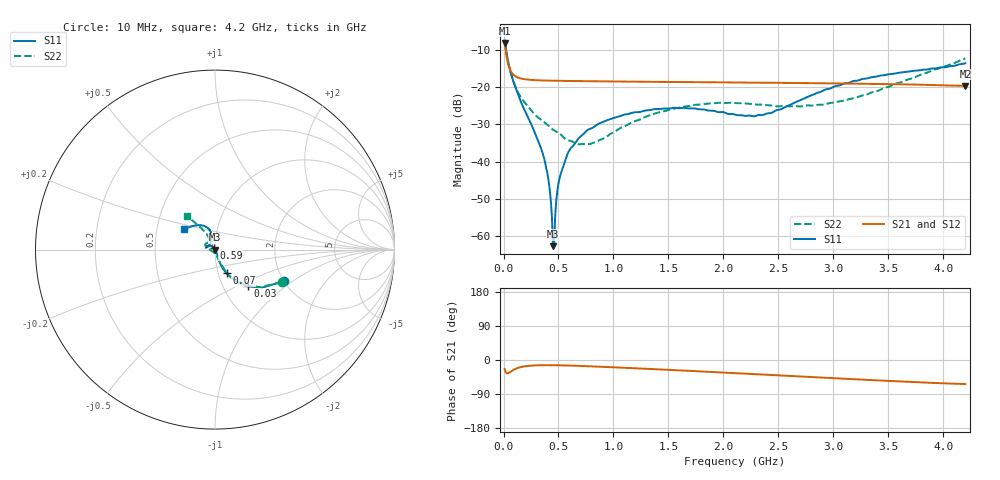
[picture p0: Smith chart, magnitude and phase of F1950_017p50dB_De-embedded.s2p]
! Integrated Device Technology
! Corporate Headquarters
! 6024 Silver Creek Valley Road
! San Jose, CA 95138  USA
! Phone:  1-408-284-8200
! Toll Free:  1-800-223-1366
! Webpage:  http://www.idt.com/
! Timing and RF Division
! 515 Groton Road, Suite 102
! Westford, MA 01886-6024
! Device:  F1950
! Description: 7-bit 0.25 dB Digital Step Attenuator
! Frequency:  150.0 -  4000.00 MHz
! Package:  4x4 mm Thin QFN Plastic Package: 24 pin
! Ports:  2 RF, 12 DC
!  Pin  1  = D0
!  Pin  2  = VDD
!  Pin  3  = Vmode
!  Pin  4  = GND
!  Pin  5  = RF1  =  Port 1
!  Pin  6  = GND
!  Pin  7  = GND
!  Pin  8  = GND
!  Pin  9  = GND
!  Pin 10  = GND
!  Pin 11  = GND
!  Pin 12  = GND
!  Pin 13  = GND
!  Pin 14  = RF2  =  Port 2
!  Pin 15  = GND
!  Pin 16  = LE
!  Pin 17  = CLK
!  Pin 18  = DATE
!  Pin 19  = D6
!  Pin 20  = D5
!  Pin 21  = D4
!  Pin 22  = D3
!  Pin 23  = D2
!  Pin 24  = D1
! State:  70
! Atten State:  17.50 dB
! Voltage:  +5.00 Volts
! Current:  Not Measured mA
! Data:  The device was measured on a the F195X evaluation board which has
!  individual transmission lines to the RF pins.  Data was collected
!  using a calibrated network analyzer.  The evaluation board was
!  de-embedded using a TRL calibration technique.
!  The reference plane is the edge of the package pin.
! Misc:  Board 2019
!  Action Tracker AT0250
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# GHz S dB R 50
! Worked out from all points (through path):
!   420 points, 10 MHz to 4.2 GHz, reference 50 ohm
!   highest |S21| = -8.20 dB at 10 MHz (marker M1); lowest = -19.7 dB at 4.2 GHz (marker M2)
!   group delay of S21, straight-line fit = 35.1 ps
!   lowest |S11| = -62.6 dB at 450 MHz (marker M3), VSWR 1.00, Z = 50.1 - j0.0332 ohm
!   |S11| at or under -10 dB: 22.86 MHz to end of sweep
!   |S22| runs from -35.4 to -7.7 dB; largest |S21 - S12| = 0.0002
!   S11 on the Smith chart (normalised r, x): 10 MHz: 1.99, -0.85; 30 MHz: 1.30, -0.57; 70 MHz: 1.10, -0.30; 590 MHz: 0.98, +0.02; 4.2 GHz: 0.69, +0.17
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0.01  -7.52 -24.8  -8.20 -23.7  -8.20 -23.7  -7.68 -26.0
0.03  -11.29 -48.2  -12.17 -35.3  -12.17 -35.3  -11.40 -48.2
0.07  -16.67 -63.9  -15.92 -29.8  -15.92 -29.8  -16.49 -62.8
0.16  -24.07 -69.7  -17.72 -18.6  -17.72 -18.5  -22.83 -69.8
0.36  -38.16 -60.0  -18.25 -13.7  -18.25 -13.7  -29.15 -76.3
0.41  -45.15 -58.3  -18.29 -13.6  -18.28 -13.6  -30.41 -77.3
0.44  -54.63 -50.1  -18.31 -13.7  -18.30 -13.7  -31.20 -80.4
0.45  -62.63 -26.6  -18.31 -13.7  -18.31 -13.7  -31.43 -81.6
0.47  -54.44 103.8  -18.32 -13.8  -18.32 -13.8  -31.79 -84.4
0.49  -47.64 115.6  -18.33 -13.9  -18.33 -13.9  -32.09 -86.4
0.51  -44.38 121.5  -18.34 -14.0  -18.34 -14.0  -32.45 -87.5
0.59  -37.43 127.3  -18.37 -14.6  -18.37 -14.6  -34.30 -99.5
0.71  -33.02 133.1  -18.42 -15.7  -18.41 -15.8  -35.31 -121.2
0.81  -30.91 137.3  -18.45 -16.9  -18.45 -16.9  -35.03 -142.6
0.99  -28.40 144.9  -18.51 -19.1  -18.51 -19.1  -32.29 -169.4
1.41  -25.88 161.7  -18.62 -24.7  -18.62 -24.7  -26.80 166.9
1.74  -25.75 167.5  -18.69 -29.3  -18.69 -29.3  -24.77 158.0
2.11  -27.43 156.3  -18.78 -34.8  -18.78 -34.8  -24.31 148.8
2.43  -26.98 123.5  -18.86 -39.4  -18.86 -39.4  -24.92 139.0
2.81  -22.12 103.3  -18.96 -45.1  -18.96 -45.2  -24.97 124.0
3.51  -16.55 116.2  -19.22 -55.3  -19.21 -55.3  -19.87 118.8
4.2  -13.64 145.6  -19.70 -63.5  -19.70 -63.6  -12.33 129.8
